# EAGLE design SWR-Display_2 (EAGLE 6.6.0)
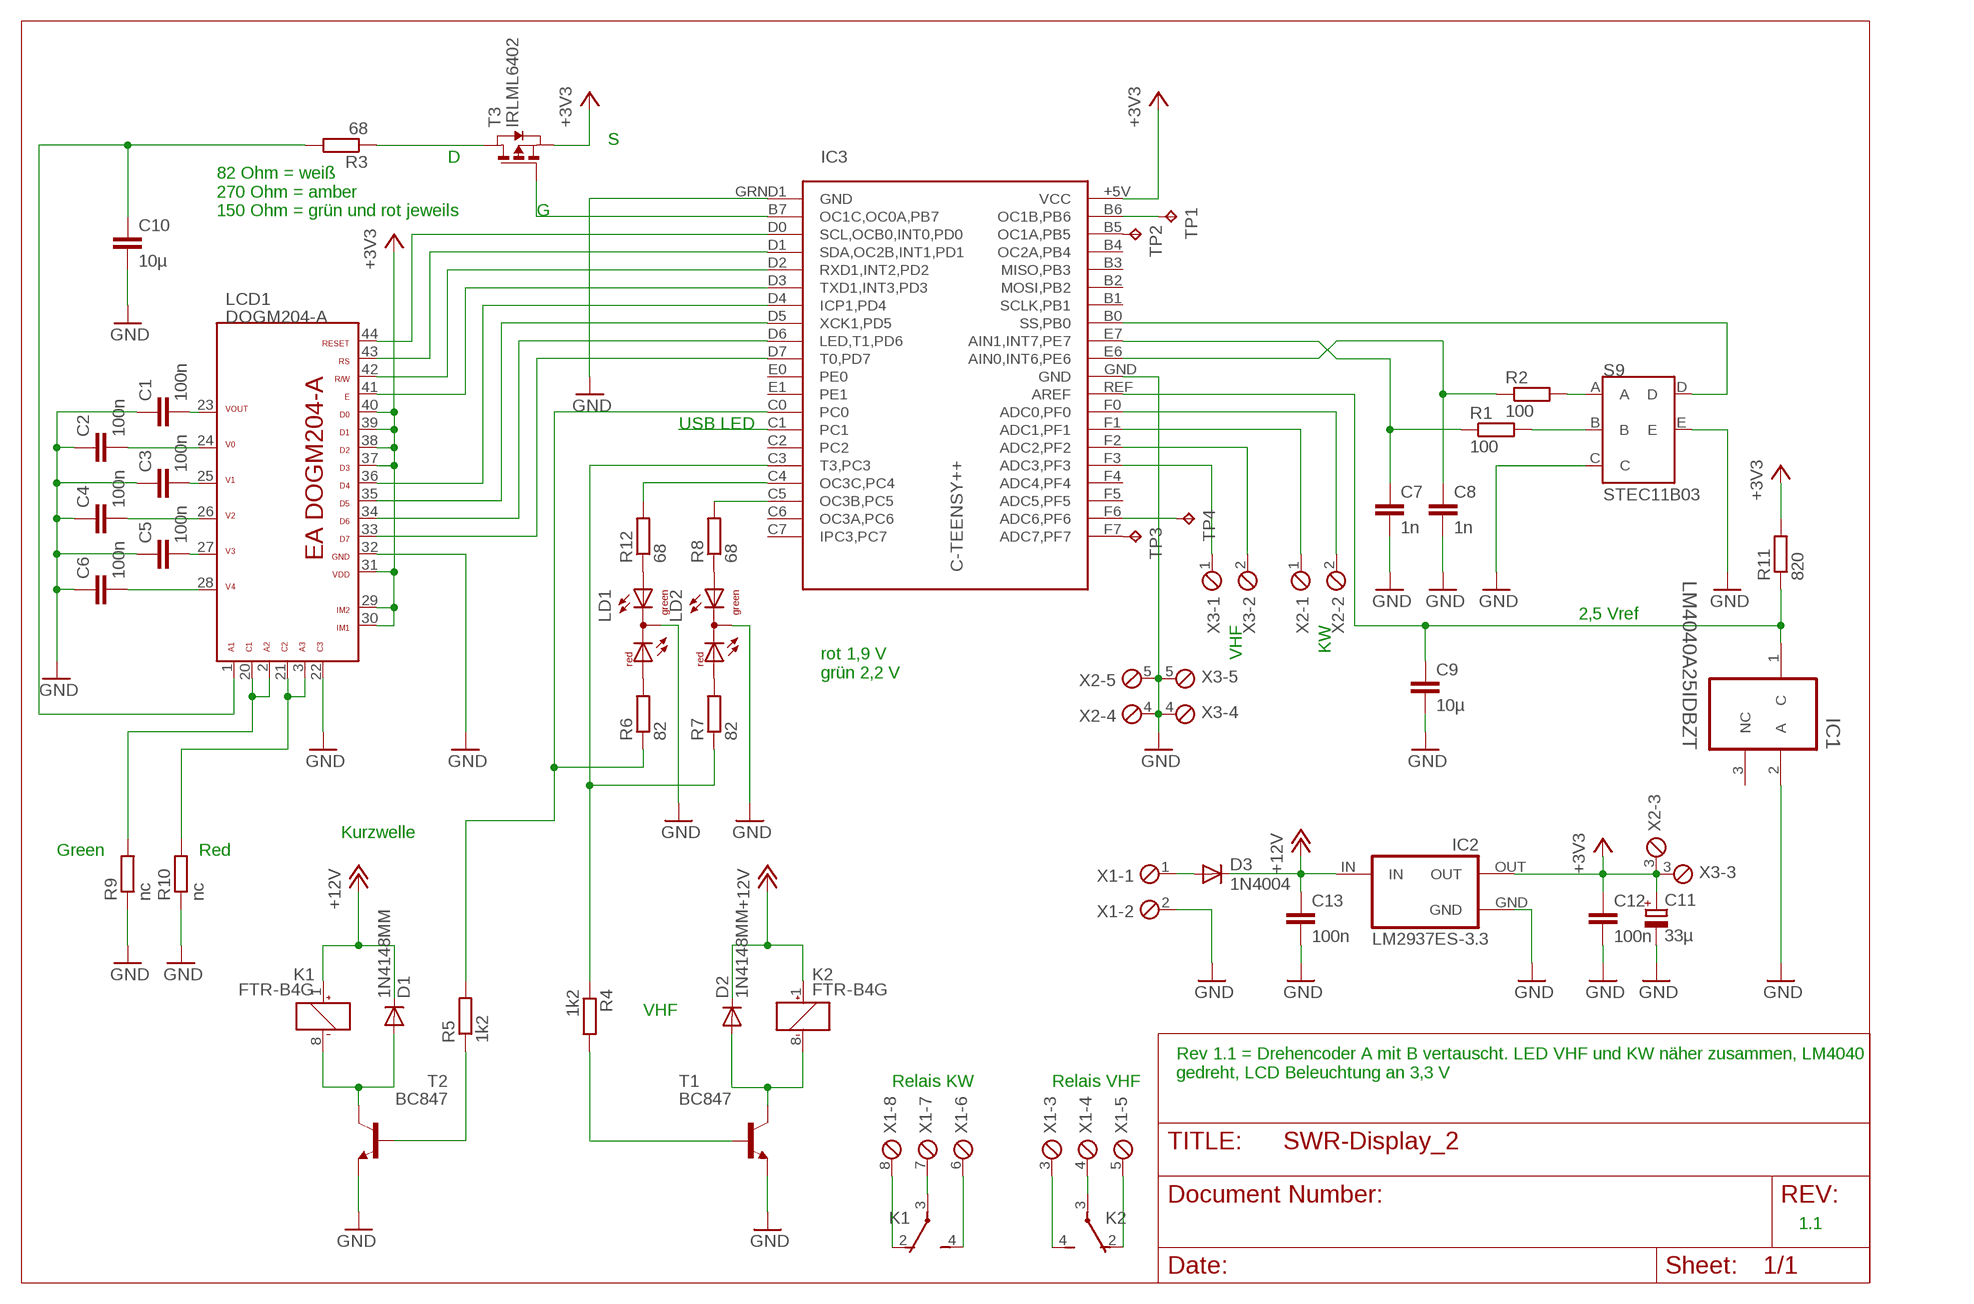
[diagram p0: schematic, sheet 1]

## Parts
C1  100n  C-EUC0805K  [C0805K]
C2  100n  C-EUC0805K  [C0805K]
C3  100n  C-EUC0805K  [C0805K]
C4  100n  C-EUC0805K  [C0805K]
C5  100n  C-EUC0805K  [C0805K]
C6  100n  C-EUC0805K  [C0805K]
C7  1n  C-EUC0805K  [C0805K]
C8  1n  C-EUC0805K  [C0805K]
C9  10µ  C-EUC0805K  [C0805K]
C10  10µ  C-EUC0805K  [C0805K]
C11  33µ  CPOL-EUD/7343-31W  [D/7343-31W]
C12  100n  C-EUC0805K  [C0805K]
C13  100n  C-EUC0805K  [C0805K]
D1  1N4148MM  [MINIMELF]
D2  1N4148MM  [MINIMELF]
D3  1N4004  [DO41-10]
IC1  LM4040A25IDBZT  LM4040A50IDBZT  [SOT95P237X112-3N]
IC2  LM2937ES-3.3  [TO263]
IC3  C-TEENSY++  [TEENSY++]
K1  FTR-B4G  [FTR-B4G]
K2  FTR-B4G  [FTR-B4G]
LCD1  DOGM204-A  [DOGM204-A]
LD1  DUOLED-RG-C  [DUOLED-C-5MM]
LD2  DUOLED-RG-C  [DUOLED-C-5MM]
R1  100  R-EU_M0805  [M0805]
R2  100  R-EU_M0805  [M0805]
R3  68  R-EU_M0805  [M0805]
R4  1k2  R-EU_M0805  [M0805]
R5  1k2  R-EU_M0805  [M0805]
R6  82  R-EU_M0805  [M0805]
R7  82  R-EU_M0805  [M0805]
R8  68  R-EU_M0805  [M0805]
R9  nc  R-EU_M0805  [M0805]
R10  nc  R-EU_M0805  [M0805]
R11  820  R-EU_M0805  [M0805]
R12  68  R-EU_M0805  [M0805]
S9  STEC11B03  ENCODER  [ENCODER]
T1  BC847  [SOT23]
T2  BC847  [SOT23]
T3  IRLML6402  [SOT-23]
TP1  TPTP20R  [TP20R]
TP2  TPTP20R  [TP20R]
TP3  TPTP20R  [TP20R]
TP4  TPTP20R  [TP20R]
X1  MPT8  [8POL254]
X2  MPT5  [5POL254]
X3  MPT5  [5POL254]

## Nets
+3V3: C11.+ C12.1 IC2.OUT IC3.+5V(VCC) LCD1.29 LCD1.30 LCD1.31 LCD1.37 LCD1.38 LCD1.39 LCD1.40 R11.2 T3.2(S) X2.3 X3.3
+12V: C13.1 D1.C D2.C D3.C IC2.IN K1.1(K:+) K2.1(K:+)
GND: C1.1 C2.1 C3.1 C4.1 C5.1 C6.1 C7.2 C8.2 C9.2 C10.2 C11.- C12.2 C13.2 IC1.2(A) IC2.GND IC3.GND IC3.GRND1(GND) LCD1.22 LCD1.32 LD1.C LD2.C R9.1 R10.1 S9.C S9.E T1.2(E) T2.2(E) X1.2 X2.4 X2.5 X3.4 X3.5
N$1: C4.2 LCD1.26
N$2: C1.2 LCD1.23
N$3: C2.2 LCD1.24
N$4: IC3.D4(ICP1,PD4) LCD1.36
N$5: IC3.D5(XCK1,PD5) LCD1.35
N$6: IC3.D6(LED,T1,PD6) LCD1.34
N$7: IC3.D7(T0,PD7) LCD1.33
N$8: IC3.D0(SCL,OCB0,INT0,PD0) LCD1.44
N$9: IC3.D1(SDA,OC2B,INT1,PD1) LCD1.43
N$10: IC3.D2(RXD1,INT2,PD2) LCD1.42
N$11: C3.2 LCD1.25
N$12: C5.2 LCD1.27
N$13: C6.2 LCD1.28
N$14: IC3.C3(T3,PC3) R4.1 R7.1
N$15: IC3.C4(OC3C,PC4) R12.2
N$16: R2.2 S9.A
N$17: R1.2 S9.B
N$18: C8.1 IC3.E6(AIN0,INT6,PE6) R2.1
N$19: C7.1 IC3.E7(AIN1,INT7,PE7) R1.1
N$20: IC3.F0(ADC0,PF0) X2.2
N$21: IC3.B0(SS,PB0) S9.D
N$22: IC3.F1(ADC1,PF1) X2.1
N$23: K2.3(-1:P) X1.4
N$24: R3.1 T3.3(D)
N$25: IC3.B7(OC1C,OC0A,PB7) T3.1(G)
N$26: C10.1 LCD1.1 R3.2
N$27: IC3.D3(TXD1,INT3,PD3) LCD1.41
N$28: LCD1.2 LCD1.20 R9.2
N$29: D1.A K1.8(K:-) T2.3(C)
N$30: R5.1 T2.1(B)
N$31: D2.A K2.8(K:-) T1.3(C)
N$32: IC3.C5(OC3B,PC5) R8.2
N$33: LD1.AR R6.2
N$34: R4.2 T1.1(B)
N$35: LD2.AR R7.2
N$36: LCD1.3 LCD1.21 R10.2
N$37: IC3.F2(ADC2,PF2) X3.2
N$38: IC3.F3(ADC3,PF3) X3.1
N$39: K2.4(-1:S) X1.3
N$40: K2.2(-1:O) X1.5
N$41: K1.2(-1:O) X1.8
N$42: K1.3(-1:P) X1.7
N$43: K1.4(-1:S) X1.6
N$44: D3.A X1.1
N$45: IC3.B6(OC1B,PB6) TP1.TP
N$46: C9.1 IC1.1(C) IC3.REF(AREF) R11.1
N$47: IC3.B5(OC1A,PB5) TP2.TP
N$48: IC3.F7(ADC7,PF7) TP3.TP
N$49: IC3.F6(ADC6,PF6) TP4.TP
N$50: LD1.AX(AG) R12.1
N$51: LD2.AX(AG) R8.1
N$53: IC3.C1
SWR_KW: IC3.C0 R5.2 R6.1
Unconnected: IC1.3(NC) IC3.B1(SCLK,PB1) IC3.B2(MOSI,PB2) IC3.B3(MISO,PB3) IC3.B4(OC2A,PB4) IC3.C2 IC3.C6(OC3A,PC6) IC3.C7(IPC3,PC7) IC3.E0 IC3.E1 IC3.F4(ADC4,PF4) IC3.F5(ADC5,PF5) K1.5(-2:S) K1.6(-2:P) K1.7(-2:O) K2.5(-2:S) K2.6(-2:P) K2.7(-2:O)

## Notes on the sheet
- S
- D
- 82 Ohm = weiß
  270 Ohm = amber
  150 Ohm = grün und rot jeweils
- G
- USB LED
- 2,5 Vref
- VHF | KW
- rot 1,9 V
  grün 2,2 V
- Kurzwelle
- Green | Red
- VHF
- Rev 1.1 = Drehencoder A mit B vertauscht. LED VHF und KW näher zusammen, LM4040 
  gedreht, LCD Beleuchtung an 3,3 V
- Relais KW | Relais VHF
- 1.1

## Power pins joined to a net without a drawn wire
GND: IC2.GND@(GND)

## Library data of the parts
C1-C6 C12 C13 = rcl:C-EU: CAPACITOR, European symbol; MF: YAGEO (PHYCOMP); MPN: CC0603MRY5V9BB104; OC_FARNELL: 431989
C7 C8 = rcl:C-EU: CAPACITOR, European symbol; MF: AVX; MPN: 06035A102JAT2A; OC_FARNELL: 317202
C9 C10 = rcl:C-EU: CAPACITOR, European symbol; MF: KEMET; MPN: C0805C106K4PACTU; OC_FARNELL: 1288204
C11 = rcl:CPOL-EU: POLARIZED CAPACITOR, European symbol
D1 D2 = RSC_IB_LIB:1N4148: DIODE; MF: MICRO COMMERCIAL COMPONENTS; MPN: DL4148-TP; OC_FARNELL: 1924344
D3 = diode:1N4004: DIODE
IC1 = LM4040:LM4040A50IDBZT: PRECISION MICROPOWER SHUNT VOLTAGE REFERENCE; MPN: LM4040A50IDBZT; OC_FARNELL: 1755108; OC_NEWARK: 58K5870; PACKAGE: 3-SOT-23; SUPPLIER: TEXAS INSTRUMENTS
IC2 = lm2937:LM2937ES-*: 400 and 500 mA Low Dropout Voltage Regulator NATIONAL SEMICONDUCTOR created by Peter.Hofmann@ph-tronic.de 10-2004 Rev.0
IC3 = teensypp:C-TEENSY++; OC_FARNELL: unknown
K1 K2 = relay:FTR-B4: ULTRA MINIATURE RELAY 2 POLES - 2 A (Slim Profile Signal Relay) FUJITSU FTR-B4 SERIES Source: FTR-B4.pdf; OC_FARNELL: unknown
LCD1 = DOGM204-A:DOGM204-A; OC_FARNELL: unknown
LD1 LD2 = led:DUOLED-RG-C: DUO LED 2 colors (red/green), 5 mm, round, common Cathode www.ligitek.com or other producers.
R1 R2 = rcl:R-EU_: RESISTOR, European symbol; MF: MULTICOMP; MPN: MC01W08055100R; OC_FARNELL: 9333703
R3-R12 = rcl:R-EU_: RESISTOR, European symbol; MF: YAGEO (PHYCOMP); MPN: RC0805FR-071R2L; OC_FARNELL: 9237135
S9 = encoder:ENCODER; OC_FARNELL: unknown
T1 T2 = RSC_IB_LIB:BC847: NPN TRANSISTOR; MF: INFINEON; MPN: BC 847C E6327; OC_FARNELL: 2432696
T3 = IRLML6402:IRLML6402; MF: INTERNATIONAL RECTIFIER; MPN: IRLML6402PBF; OC_FARNELL: 9103503
TP1-TP4 = testpad:TP: Test pad
X1 = con-phoenix-254:MPT8: PHOENIX CONNECTOR; OC_FARNELL: unknown; OC_NEWARK: unknown
X2 X3 = con-phoenix-254:MPT5: PHOENIX CONNECTOR; OC_FARNELL: unknown; OC_NEWARK: unknown

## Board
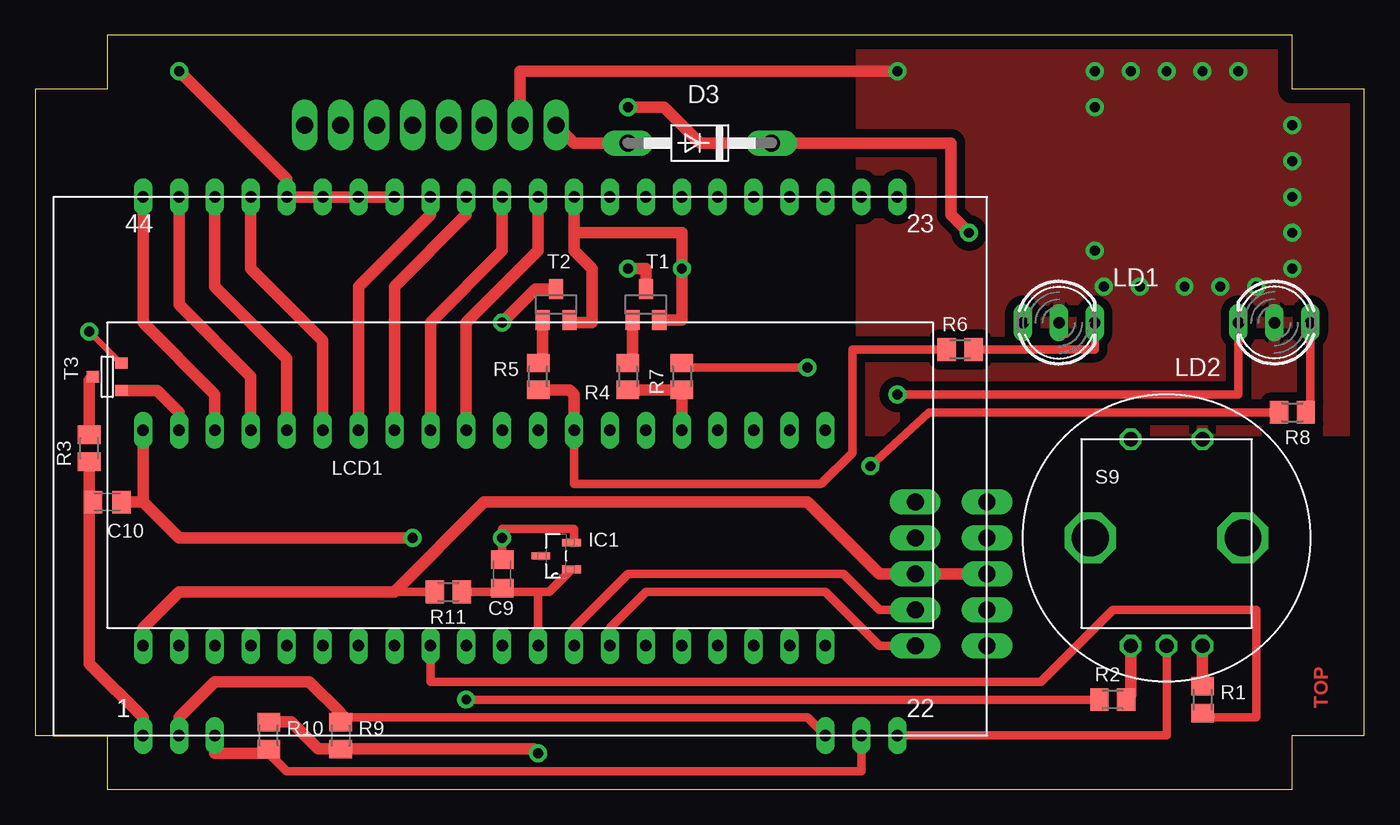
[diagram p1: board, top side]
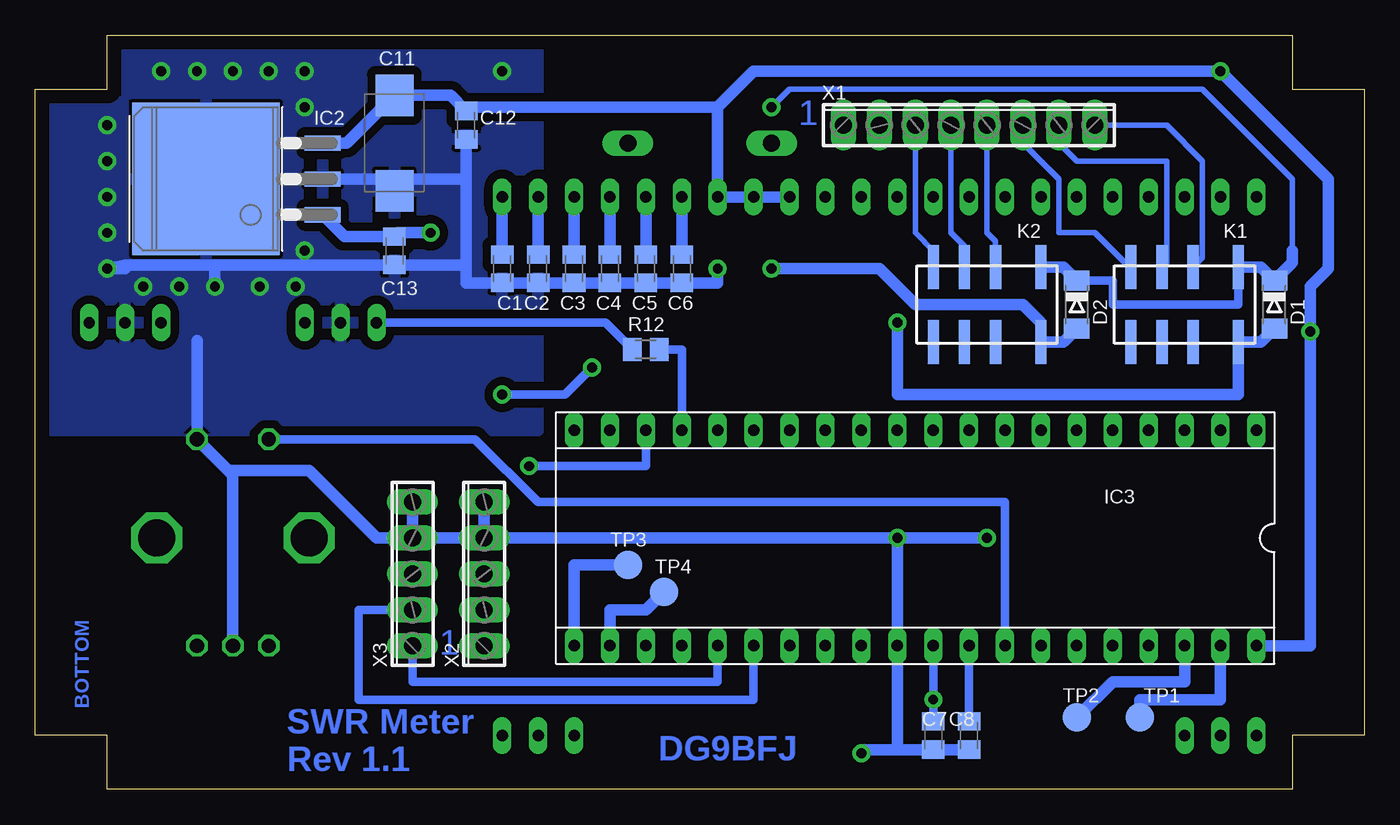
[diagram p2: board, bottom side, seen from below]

Size 93.98 x 53.34 mm. Coordinates in mm from the lower left corner, seen from the top.
Outline: 5.08,0 88.9,0 88.9,3.81 93.98,3.81 93.98,49.53 88.9,49.53 88.9,53.34 5.08,53.34 5.08,49.53 0,49.53 0,3.81 5.08,3.81 5.08,0
Copper layers (1*16): Top 0.035mm / dielectric 1.5mm / Bottom 0.035mm
Design rules "Bilex DRU": minimum track width 10mil, minimum drill 24mil, track to track 10mil, track to pad 10mil, pad to pad 10mil, via to via 10mil, smd to smd 10mil, copper to edge 40mil, drill to drill 8mil, minimum pad ring 10mil, minimum via ring 8mil, stop-mask expansion 4mil, vias tented up to drill 0mil, thermal gap 10mil

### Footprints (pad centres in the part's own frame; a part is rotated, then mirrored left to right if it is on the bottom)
C0805K = smd 1.3 x 1.6: 1 -1,0; 2 1,0
D/7343-31W = smd 2.95 x 2.7: + 3.375,0; - -3.375,0
MINIMELF = smd 1.4 x 1.8: A 1.7,0; C -1.7,0
DO41-10 = drill 1.2 pad 1.676 long: A 5.08,0; C -5.08,0
SOT95P237X112-3N = smd 1.321 x 0.559: 1 -1.092,0.94; 2 -1.092,-0.94 | smd 1.321 x 0.508: 3 1.092,0
TO263 = smd 1.067 x 2.54: GND 0,0; IN -2.54,0; OUT 2.54,0 | smd 10.795 x 10.414: GND@ 0,8.255
TEENSY++ = drill 0.813 long: +5V -24.13,7.62; B0 -6.35,7.62; B1 -8.89,7.62; B2 -11.43,7.62; B3 -13.97,7.62; B4 -16.51,7.62; B5 -19.05,7.62; B6 -21.59,7.62; B7 -21.59,-7.62; C0 6.35,-7.62; C1 8.89,-7.62; C2 11.43,-7.62; C3 13.97,-7.62; C4 16.51,-7.62; C5 19.05,-7.62; C6 21.59,-7.62; C7 24.13,-7.62; D0 -19.05,-7.62; D1 -16.51,-7.62; D2 -13.97,-7.62; D3 -11.43,-7.62; D4 -8.89,-7.62; D5 -6.35,-7.62; D6 -3.81,-7.62; D7 -1.27,-7.62; E0 1.27,-7.62; E1 3.81,-7.62; E6 -1.27,7.62; E7 -3.81,7.62; F0 6.35,7.62; F1 8.89,7.62; F2 11.43,7.62; F3 13.97,7.62; F4 16.51,7.62; F5 19.05,7.62; F6 21.59,7.62; F7 24.13,7.62; GND -24.13,-7.62; GRND1 1.27,7.62; REF 3.81,7.62
FTR-B4G = smd 0.8 x 3.1: 1 -3.8,-2.65; 2 -0.6,-2.65; 3 1.6,-2.65; 4 3.8,-2.65; 5 3.8,2.65; 6 1.6,2.65; 7 -0.6,2.65; 8 -3.8,2.65
DOGM204-A = drill 0.813 long: 1 -25.4,-21.59; 2 -22.86,-21.59; 3 -20.32,-21.59; 20 22.86,-21.59; 21 25.4,-21.59; 22 27.94,-21.59; 23 27.94,16.51; 24 25.4,16.51; 25 22.86,16.51; 26 20.32,16.51; 27 17.78,16.51; 28 15.24,16.51; 29 12.7,16.51; 30 10.16,16.51; 31 7.62,16.51; 32 5.08,16.51; 33 2.54,16.51; 34 0,16.51; 35 -2.54,16.51; 36 -5.08,16.51; 37 -7.62,16.51; 38 -10.16,16.51; 39 -12.7,16.51; 40 -15.24,16.51; 41 -17.78,16.51; 42 -20.32,16.51; 43 -22.86,16.51; 44 -25.4,16.51
DUOLED-C-5MM = drill 0.813 long: AR 2.54,0; AX -2.54,0; C 0,0
M0805 = smd 1.3 x 1.6: 1 -0.95,0; 2 0.95,0
ENCODER = drill 1 octagon: A -2.54,-7.62; B 2.54,-7.62; C 0,-7.62; D -2.54,6.985; E 2.54,6.985 | drill 2.6 octagon: P$1 5.397,0; P$2 -5.397,0
SOT23 = smd 1 x 1.4: 1 -0.95,-1.1; 2 0.95,-1.1; 3 0,1.1
SOT-23 = smd 0.787 x 0.889: 1 0.991,1.016; 2 -0.94,1.016; 3 0.025,-1.016
TP20R = smd 2 x 2: TP 0,0
8POL254 = drill 1.2 long: 1 -8.89,0; 2 -6.35,0; 3 -3.81,0; 4 -1.27,0; 5 1.27,0; 6 3.81,0; 7 6.35,0; 8 8.89,0
5POL254 = drill 1.2 long: 1 -5.08,0; 2 -2.54,0; 3 0,0; 4 2.54,0; 5 5.08,0

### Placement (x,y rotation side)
C1  60.96,36.83 90 bottom
C2  58.42,36.83 90 bottom
C3  55.88,36.83 90 bottom
C4  53.34,36.83 90 bottom
C5  50.8,36.83 90 bottom
C6  48.26,36.83 90 bottom
C7  27.94,3.81 270 bottom
C8  30.48,3.81 270 bottom
C9  33.02,15.24 90 top
C10  5.08,20.32 0 top
C11  68.58,45.72 90 bottom
C12  63.5,46.99 270 bottom
C13  68.58,38.1 270 bottom
D1  6.35,34.29 270 bottom
D2  20.32,34.29 270 bottom
D3  46.99,45.72 180 top
IC1  36.83,16.51 180 top
IC2  73.66,43.18 90 bottom
IC3  31.75,17.78 180 bottom
K1  12.7,34.29 180 bottom
K2  26.67,34.29 180 bottom
LCD1  33.02,25.4 0 top
LD1  72.39,33.02 0 top
LD2  87.63,33.02 180 top
R1  82.55,6.35 90 top
R2  76.2,6.35 0 top
R3  3.81,24.13 270 top
R4  41.91,29.21 90 top
R5  35.56,29.21 270 top
R6  65.41,31.11 0 top
R7  45.72,29.21 90 top
R8  88.9,26.67 180 top
R9  21.59,3.81 90 top
R10  16.51,3.81 270 top
R11  29.21,13.97 180 top
R12  50.8,31.11 0 bottom
S9  80.01,17.78 0 top
T1  43.18,34.29 0 top
T2  36.83,34.29 0 top
T3  5.08,29.21 270 top
TP1  15.88,5.08 0 bottom
TP2  20.32,5.08 0 bottom
TP3  52.07,15.88 0 bottom
TP4  49.53,13.97 0 bottom
X1  27.94,46.99 0 bottom
X2  62.23,15.24 90 bottom
X3  67.31,15.24 90 bottom

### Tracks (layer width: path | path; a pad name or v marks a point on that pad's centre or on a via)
+3V3  (via drill 0.7 pad 1.27)
  Top 0.406: T3.2 6.04,30.15 v3.81,32.38
  Top 0.61: R11.2 25.4,13.97
  Top 0.813: LCD1.37 LCD1.38 LCD1.39 LCD1.40 17.78,43.18 v10.16,50.8 | IC3.+5V 7.62,11.43 10.16,13.97 25.4,13.97 31.75,20.32 54.61,20.32 59.69,15.24 X2.3 X3.3
  Bottom 0.813: LCD1.31 LCD1.30 LCD1.29 45.72,48.26 | IC3.+5V 3.81,10.16 v3.81,32.38 3.81,33.66 3.81,35.56 2.54,36.83 2.54,43.18 v10.16,50.8 43.18,50.8 45.72,48.26 | IC2.OUT 71.95,45.72 C11.+ 64.61,49.09 C12.1 63.5,48.26 45.72,48.26
+12V  (via drill 0.7 pad 1.27)
  Top 0.813: v66.04,39.37 64.77,40.64 64.77,45.72 D3.C 46.99,45.72 44.45,48.26 v41.91,48.26
  Bottom 0.406: 5.08,38.1 5.08,43.18 11.43,49.53 40.64,49.53 v41.91,48.26
  Bottom 0.61: D2.C 17.78,35.99 17.78,34.29 8.9,34.29 | 8.89,34.29 8.9,34.29 | 8.9,34.29 K1.1
  Bottom 0.813: K1.1 7.3,36.94 D1.C 5.08,37.26 5.08,38.1 | K2.1 21.27,36.94 D2.C | v66.04,39.37 68.31,39.37 C13.1 72.12,39.1 IC2.IN
GND  (via drill 0.7 pad 1.27)
  Top 0.61: LCD1.22 80.01,3.81 S9.C | 33.02,16.18 C9.2 v33.02,17.78 33.02,18.41 38.1,18.41 38.1,17.45 IC1.2
  Top 0.813: R10.1 18.1,4.76 20,2.86 R9.1 35.24,2.86 v35.56,2.54 | LCD1.32 38.1,39.37 | 38.1,39.37 38.1,38.1 39.37,36.83 39.37,33.02 37.95,33.02 T2.2 | T1.2 45.72,33.19 v45.72,36.83 45.72,39.37 38.1,39.37 | C10.2 7.62,20.32 | X1.2 34.29,50.8 v60.96,50.8 | IC3.GND 7.62,20.32 | 7.62,20.32 10.16,17.78 v26.67,17.78
  Bottom 0.813: C7.2 C8.2 33.02,2.81 | 33.02,2.81 IC3.GRND1 v33.02,17.78 | S9.C 80.01,22.23 80.33,22.54 | 80.33,22.54 S9.E 82.55,31.75 | 63.5,37.1 63.5,35.83 C1.1 C2.1 C3.1 C4.1 C5.1 C6.1 45.72,35.83 v45.72,36.83 | 63.5,37.1 C13.2 81.28,37.1 | 81.28,37.1 87.63,37.1 v88.9,36.83 87.63,36.83 | IC2.GND@ IC2.GND 68.58,43.18 | v35.56,2.54 35.29,2.81 33.02,2.81 | 68.58,43.18 C11.- | C12.2 63.5,43.18 | 63.5,43.18 63.5,37.1 | 68.58,43.18 63.5,43.18 | 80.33,22.54 74.61,22.54 69.85,17.78 X3.4 | v26.67,17.78 v33.02,17.78 | X3.4 X2.4 | v33.02,17.78 X2.4 | X2.5 X2.4 | X3.5 X3.4 | v81.28,35.56 81.28,37.1
  other vias: 74.93,50.8 77.47,50.8 80.01,50.8 82.55,50.8 85.09,50.8 88.9,46.99 88.9,44.45 88.9,41.91 88.9,39.37 86.36,35.56 83.82,35.56 78.11,35.56 75.56,35.56 74.93,38.1 74.93,48.26
  pour Bottom (isolate 0.61): 58.42,53.34 58.42,25.4 93.98,25.4 93.98,49.53 88.9,49.53 88.9,53.34
  pour Top (isolate 0.61): 58.42,53.34 58.42,25.4 93.98,25.4 93.98,49.53 88.9,49.53 88.9,53.34
N$1
  Bottom 0.813: LCD1.26 C4.2
N$2
  Bottom 0.813: LCD1.23 C1.2
N$3
  Bottom 0.813: LCD1.24 C2.2
N$4
  Top 0.813: LCD1.36 27.94,40.64 22.86,35.56 IC3.D4
N$5
  Top 0.813: IC3.D5 25.4,35.56 30.48,40.64 LCD1.35
N$6
  Top 0.813: LCD1.34 33.02,38.1 27.94,33.02 IC3.D6
N$7
  Top 0.813: LCD1.33 35.56,38.1 30.48,33.02 IC3.D7
N$8
  Top 0.813: LCD1.44 7.62,33.02 12.7,27.94 IC3.D0
N$9
  Top 0.813: IC3.D1 15.24,29.21 10.16,34.29 LCD1.43
N$10
  Top 0.813: LCD1.42 12.7,35.56 17.78,30.48 IC3.D2
N$11
  Bottom 0.813: LCD1.25 C3.2
N$12
  Bottom 0.813: LCD1.27 C5.2
N$13
  Bottom 0.813: LCD1.28 C6.2
N$14
  Top 0.813: R4.1 R7.1 IC3.C3
N$15
  Bottom 0.61: R12.2 48.26,31.11 IC3.C4
N$16
  Top 0.813: S9.A 77.47,6.67 R2.2
N$17
  Top 0.813: R1.2 S9.B
N$18  (via drill 0.7 pad 1.27)
  Top 0.61: v30.48,6.35 R2.1
  Bottom 0.61: IC3.E6 v30.48,6.35 C8.1
N$19
  Top 0.61: 82.87,5.4 R1.1 82.55,5.08 86.36,5.08 86.36,12.7 76.2,12.7 71.12,7.62 27.94,7.62 IC3.E7
  Bottom 0.61: C7.1 IC3.E7
N$20
  Top 0.61: IC3.F0 38.1,11.43 41.91,15.24 57.15,15.24 59.69,12.7 X2.2
N$21
  Bottom 0.61: IC3.B0 25.4,20.32 58.42,20.32 62.87,24.77 S9.D
N$22
  Top 0.61: IC3.F1 40.64,11.43 43.18,13.97 55.88,13.97 59.69,10.16 X2.1
N$23
  Bottom 0.406: K2.3 28.27,38.43 29.21,39.37 X1.4
N$24
  Top 0.813: R3.1 3.81,28.93 T3.3
N$25
  Top 0.813: T3.1 8.61,28.22 10.16,26.67 IC3.B7
N$26
  Top 0.813: 3.81,20.32 3.81,8.89 7.62,5.08 LCD1.1 | 3.81,20.32 R3.2 | C10.1 3.81,20.32
N$27
  Top 0.813: IC3.D3 20.32,31.75 15.24,36.83 LCD1.41
N$28
  Top 0.61: LCD1.20 54.61,5.08 21.91,5.08
  Top 0.813: LCD1.2 10.16,5.08 12.7,7.62 15.24,7.62 19.37,7.62 21.59,5.4 R9.2 21.91,5.08
N$29  (via drill 0.7 pad 1.27)
  Top 0.813: v33.02,33.02 35.39,35.39 T2.3
  Bottom 0.813: D1.A 7.3,31.64 K1.8 8.89,27.94 33.02,27.94 v33.02,33.02
N$30
  Top 0.813: T2.1 35.88,30.48 R5.1
N$31  (via drill 0.7 pad 1.27)
  Top 0.813: v41.91,36.83 43.01,36.83 43.18,36.83 T1.3
  Bottom 0.813: D2.A 21.27,31.64 K2.8 22.87,33.03 24.13,34.29 31.75,34.29 34.29,36.83 v41.91,36.83
N$32  (via drill 0.7 pad 1.27)
  Top 0.61: R8.2 63.19,26.67 v59.05,22.86
  Bottom 0.61: v59.05,22.86 50.8,22.86 IC3.C5
N$33
  Top 0.61: R6.2 74.93,31.11 LD1.AR
N$34
  Top 0.61: 42.23,30.48 41.91,30.48 R4.2
  Top 0.813: T1.1 42.23,30.48
N$35  (via drill 0.7 pad 1.27)
  Top 0.61: R7.2 46.03,29.84 v54.61,29.84 | LD2.AR 85.09,27.94 v60.96,27.94
  Bottom 0.61: v60.96,27.94 56.52,27.94 v54.61,29.84
N$36
  Top 0.61: LCD1.21 58.42,1.27 17.78,1.27 16.51,2.54
  Top 0.813: LCD1.3 12.7,2.54 16.51,2.54 R10.2
N$37
  Bottom 0.61: IC3.F2 43.18,6.35 71.12,6.35 71.12,12.7 X3.2
N$38
  Bottom 0.61: IC3.F3 45.72,7.62 67.31,7.62 X3.1
N$39
  Bottom 0.406: K2.4 30.47,38.09 31.75,39.37 X1.3
N$40
  Bottom 0.406: K2.2 26.07,38.77 26.67,39.37 X1.5
N$41
  Bottom 0.406: K1.2 11.43,37.61 11.43,44.45 13.97,46.99 X1.8
N$42
  Bottom 0.406: K1.3 13.97,37.27 13.97,44.45 20.32,44.45 21.59,45.72 X1.7
N$43
  Bottom 0.406: X1.6 24.13,45.72 21.59,43.18 21.59,39.37 19.05,39.37 16.62,36.94 K1.4
N$44
  Top 0.813: X1.1 38.1,45.72 D3.A
N$45
  Bottom 0.813: TP1.TP 15.88,6.35 10.16,6.35 IC3.B6
N$46
  Top 0.61: R11.1 33.02,13.97 C9.1 33.29,13.97 35.56,13.97 | IC1.1 36.32,13.97 35.56,13.97 | IC3.REF 35.56,13.97
N$47
  Bottom 0.813: TP2.TP 17.78,7.62 12.7,7.62 IC3.B5
N$48
  Bottom 0.813: TP3.TP 55.24,15.88 55.88,15.88 IC3.F7
N$49
  Bottom 0.813: TP4.TP 50.8,12.7 53.34,12.7 IC3.F6
N$50
  Bottom 0.61: R12.1 53.66,33.02 LD1.AX
N$51
  Top 0.61: R8.1 90.17,26.99 LD2.AX
SWR_KW
  Top 0.61: R6.1 57.78,31.11 57.78,23.81 55.56,21.59 38.1,21.59 IC3.C0
  Top 0.813: IC3.C0 38.1,27.94 37.78,28.26 R5.2

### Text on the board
Top: TOP
Bottom: 1 | 1 | BOTTOM | DG9BFJ | SWR Meter / Rev 1.1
